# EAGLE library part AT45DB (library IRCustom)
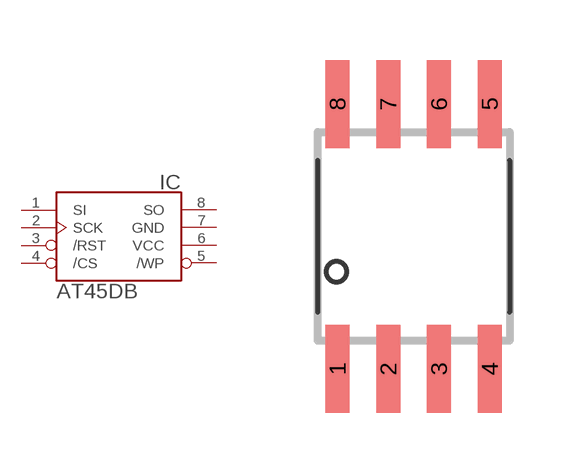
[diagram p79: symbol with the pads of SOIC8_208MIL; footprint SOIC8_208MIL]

Designator prefix IC

## AT45DB-S  [SOIC8_208MIL]
1  SI  in
2  SCK  in
3  /RST  in
4  /CS  in
5  /WP  in
6  VCC  pwr
7  GND  pwr
8  SO  out

## Footprint SOIC8_208MIL (pad centres in mm)
Small Outline IC - 208mil Wide
smd 0.6 x 2.2: 1 -1.905,-3.315; 2 -0.635,-3.315; 3 0.635,-3.315; 4 1.905,-3.315; 5 1.905,3.315; 6 0.635,3.315; 7 -0.635,3.315; 8 -1.905,3.315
